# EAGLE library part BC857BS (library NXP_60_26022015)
PNP double transistor in an SC-88; SOT363 plastic package. AAL Eindhoven MK
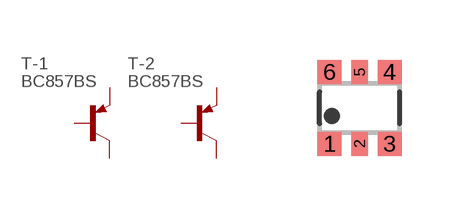
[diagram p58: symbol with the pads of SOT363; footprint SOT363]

Designator prefix T; gates -1=PNP -2=PNP

## BC857BS  [SOT363]
1  -1:E  pas
2  -1:B  pas
3  -2:C  pas
4  -2:E  pas
5  -2:B  pas
6  -1:C  pas

## Footprint SOT363 (pad centres in mm)
SOT363 Plastic surface-mounted package; 6 leads JEDEC: -- IEC: -- JEITA: SC-88
smd 0.6 x 0.6: 1 -0.75,-0.9; 3 0.75,-0.9; 4 0.75,0.9; 6 -0.75,0.9
smd 0.4 x 0.6: 2 0,-0.9; 5 0,0.9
